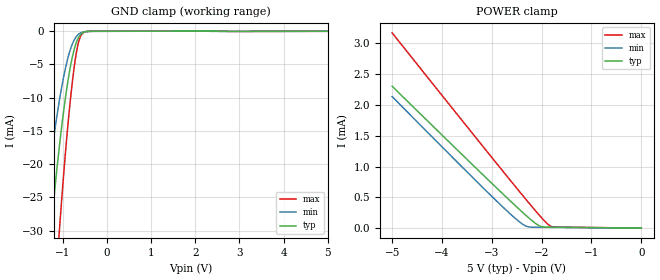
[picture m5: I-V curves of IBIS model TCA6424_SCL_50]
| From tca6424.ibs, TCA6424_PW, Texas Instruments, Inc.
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[Model]   TCA6424_SCL_50
Model_type  Input
Vinl=1.35
Vinh=3.85
| variable   typ   min   max
C_comp   2.12pF   1.76pF   2.26pF
[Temperature Range]   40   100   -40
| Ambient temperature   25   85   -40
[Voltage range]   5   4.5   5.5
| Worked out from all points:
|   GND clamp passes 1 mA (typ) near -0.65 V on its own axis
|   POWER clamp passes 1 mA (typ) near -3.35 V on its own axis
[GND Clamp]
| TCA6424_SCL_50
|   Voltage   I(typ)   I(min)   I(max)
-5V       -421.5mA   -327.2mA   -555.2mA
-1.48V    -46.19mA   -30.98mA   -72.8mA
-1.435V   -42.58mA   -28.34mA   -67.61mA
-1.265V   -29.77mA   -19.11mA   -48.89mA
-1.085V   -17.96mA   -10.85mA   -30.98mA
-1.05V    -15.92mA   -9.467mA   -27.79mA
-930mV    -9.667mA   -5.361mA   -17.73mA
-795mV    -4.311mA   -2.158mA   -8.467mA
-680mV    -1.503mA   -712.6uA   -2.841mA
-585mV    -421uA     -217.3uA   -621uA
-310mV    -3.791uA   -3.288uA   -3.906uA
5V        572.5pA    3.503uA    -5.522uA
[POWER Clamp]
| TCA6424_SCL_50
|   Voltage   I(typ)   I(min)   I(max)
-5V       2.303mA    2.136mA    3.169mA
-3.24V    914.9uA    706.8uA    1.389mA
-2.49V    336.9uA    132.2uA    639.2uA
-2.3V     197.1uA    30.18uA    452.5uA
-2.08V    54.82uA    14.6uA     241.4uA
-1.99V    23.08uA    13.94uA    159uA
-1.86V    16.46uA    13.03uA    54.56uA
-1.805V   15.92uA    12.64uA    27.89uA
-1.735V   15.3uA     12.15uA    19.51uA
-84.45fV  572.5pA    1.628nA    108.3pA
